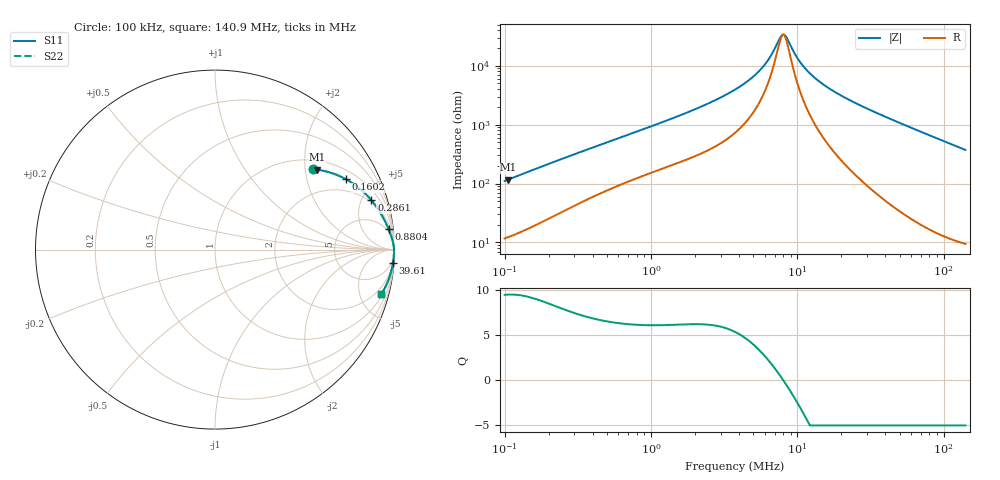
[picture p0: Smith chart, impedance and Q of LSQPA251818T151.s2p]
! LSQPA251818T151  S-PARAMETER MODEL  ( General Type )
! Model Generated by TAIYO YUDEN Corporation (http://www.ty-top.com)
! Version 3.0
! TAIYO YUDEN Control No. 160907NF25SB-FAC
! Copyright(c) 2007 TAIYO YUDEN CO.,LTD. All Rights Reserved.
! Product Description (link to TY-COMPAS)
! https://ds.yuden.co.jp/TYCOMPAS/or/detail?pn=LSQPA251818T151K&u=M
! Products Name : Inductors
! Characteristics :
!  Inductance : 150 uH , SRF(min) : 7.0 MHz , DC Resistance(max) : 7.93 Ohm
!  Rated Current : Saturation :140 mA , Temp Rise : 130 mA (40 degC)
!  Case Size : 2.5 x 1.8 / 0.098 x 0.071 [mm/inch] , Thickness : 1.8 / 0.071 [mm/inch]
!  (Conditions: Temperature = 25 degC , DC Bias Current/Voltage = 0A / 0V)
! External Node Assignments :
!  1  o---GGG---o  2
! GND o---------o GND
! Frequency Range : 0.1MHz  -  140.89697MHz  [ 402 STEP ]
# MHz S RI R 50
! Freq[MHz].  S11 Real  S11 Imag  S21 Real  S21 Imag  S12 Real  S12 Imag  S22 Real  S22 Imag
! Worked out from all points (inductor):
!   401 points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, 100 kHz to 140.9 MHz, reference 50 ohm
!   read as one part in series: L = 174 uH near 103.7 kHz
!   highest Q = 9.45 at 105.6 kHz (marker M1), where L = 175 uH
!   self-resonance near 7.892 MHz
!   S11 on the Smith chart (normalised r, x): 100 kHz: 1.23, +2.20; 160.2 kHz: 1.38, +3.47; 286.1 kHz: 1.79, +5.96; 880.4 kHz: 4, +16; 39.61 MHz: 2, -27; 140.9 MHz: 1.19, -7.43
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0.1  0.5447 0.4478  0.4553 -0.4478  0.4553 -0.4478  0.5447 0.4478
0.105589  0.5684 0.4452  0.4316 -0.4452  0.4316 -0.4452  0.5684 0.4452
0.160206  0.7306 0.3916  0.2694 -0.3916  0.2694 -0.3916  0.7306 0.3916
0.286148  0.8712 0.2751  0.1288 -0.2751  0.1288 -0.2751  0.8712 0.2751
0.336853  0.8953 0.2442  0.1047 -0.2442  0.1047 -0.2442  0.8953 0.2442
0.880381  0.9677 0.1128  0.0323 -0.1128  0.0323 -0.1128  0.9677 0.1128
1.134703  0.9763 0.0905  0.0237 -0.0905  0.0237 -0.0905  0.9763 0.0905
2.300912  0.9904 0.0458  0.00961 -0.0458  0.00961 -0.0458  0.9904 0.0458
3.753625  0.9947 0.0247  0.00528 -0.0247  0.00528 -0.0247  0.9947 0.0247
4.751056  0.9959 0.0164  0.00414 -0.0164  0.00414 -0.0164  0.9959 0.0164
5.695248  0.9964 0.0105  0.00355 -0.0105  0.00355 -0.0105  0.9964 0.0105
6.584013  0.9968 0.006  0.00322 -0.006  0.00322 -0.006  0.9968 0.006
7.611473  0.997 0.00158  0.003 -0.00158  0.003 -0.00158  0.997 0.00158
8.036843  0.9971 -7.36e-05  0.00293 7.36e-05  0.00293 7.36e-05  0.9971 -7.36e-05
8.485985  0.9971 -0.00173  0.00288 0.00173  0.00288 0.00173  0.9971 -0.00173
9.634031  0.9972 -0.00562  0.00281 0.00562  0.00281 0.00562  0.9972 -0.00562
10.54798  0.9972 -0.00845  0.00279 0.00845  0.00279 0.00845  0.9972 -0.00845
12.64421  0.9972 -0.0144  0.00283 0.0144  0.00283 0.0144  0.9972 -0.0144
19.53556  0.9965 -0.0309  0.0035 0.0309  0.0035 0.0309  0.9965 -0.0309
39.61356  0.992 -0.072  0.00795 0.072  0.00795 0.072  0.992 -0.072
42.59248  0.9911 -0.0777  0.00888 0.0777  0.00888 0.0777  0.9911 -0.0777
140.897  0.9271 -0.2476  0.0729 0.2476  0.0729 0.2476  0.9271 -0.2476
